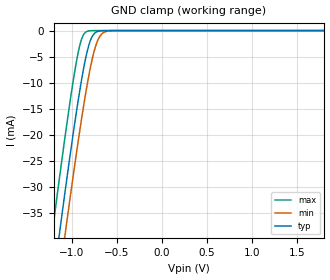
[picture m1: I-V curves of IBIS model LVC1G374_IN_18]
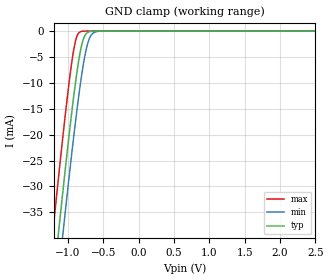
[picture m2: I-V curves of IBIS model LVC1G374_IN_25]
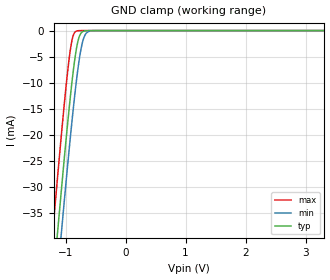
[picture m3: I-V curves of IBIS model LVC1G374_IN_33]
| TEXAS INSTRUMENTS INCORPORATED
| Standard Linear and Logic Group
| IBIS Model of SN74LVC1G374
| Single D-Type Flip-Flop with 3-State Output
| This file contains package information for the following:
|  SOT 6-pin (DBV) package as [Component] LVC1G374_DBV
|  SOT 6-pin (DCK) package as [Component] LVC1G374_DCK
|  DSBGA 6-pin (YEP) package as [Component] LVC1G374_YEP
|  DSBGA 6-pin (YZP) package as [Component] LVC1G374_YZP
| This device can be powered at the following Vccs:
|  1.8 volt Vcc
|  2.5 volt Vcc
|  3.3 volt Vcc
|  5 volt Vcc
| This file provides unique models under the [Model Selector] for each Vcc.
| For operation at a specific Vcc, select the appropriate model after each
| [Model Selector] keyword.
[IBIS Ver]   3.2
[Comment char]  |_char
[File Name]   sn74lvc1g374.ibs
[File Rev]   1.2 | x_die
[Date]   May 27, 2003
[Source]   Data created from TI-SPICE simulations at TI-SLL.
[Notes]   The following is an IBIS list for the LVC1G374.
   Please contact sllibis@ti.com with questions and
   comments concerning SLL IBIS models.
   - FILE REV HISTORY
   - 1.2 YEP and YZP packages released on 05/27/04
   - Due to the fact that the Device is 5.5-V Input tolarent,
   the pulldown model has some Non-Monotonic Warnings.
   - Power clamp data deleted as there is no power-clamp diode.
[Disclaimer] Property of Texas Instruments Incorporated.  Unauthorized
   reproduction and/or distribution is strictly prohibited.
   This product is protected under copyright law.
   Created  2003, (C) Copyright  2003, Texas Instruments
   Incorporated, All Rights Reserved
   UNLESS THERE IS A SIGNED, WRITTEN AGREEMENT TO THE
   CONTRARY, TEXAS INSTRUMENTS (TI) IS PROVIDING THE IBIS
   MODELS  AND WITHOUT ANY WARRANTY, EXPRESSED OR
   IMPLIED.  TI assumes no liability for:
   1) the accuracy of the IBIS models provided to your
   company;
   2) the proper functioning of these IBIS Models in your
   design or for any resulting applications; or
   3) infringement of patents, copyrights or intellectual
   property rights resulting from your use of these IBIS
   models.
   TI provides IBIS Models as a service to our customers.
   You and your company shall not distribute, sell or give
   these models to anyone else without prior written
   permission from TI.
   TI reserves the right to make changes to our products or
   to discontinue any semiconductor product or service
   without notice, and advises our customers to obtain the
   latest version of relevant information to verify, before
   placing orders, that the information being relied on is
   current.
   Please be aware that your receipt and use of the IBIS
   information provided shall serve as acceptance of these
   terms and conditions.  If you do not accept these terms,
   you should return or destroy the IBIS models and any
   other accompanying information immediately.
| Component LVC1G374_DBV 6-pin SOT
[Component]   LVC1G374_DBV
[Manufacturer]   Texas Instruments, Inc.
[Package]
|   typ   min   max
R_pkg   2.500e-02   1.900e-02   3.700e-02
L_pkg   1.524e-09   1.260e-09   1.751e-09
C_pkg   2.450e-13   1.980e-13   2.640e-13
[Pin]   signal_name   model_name   R_pin   L_pin   C_pin
1   CLK   LVC1G374_IN   2.100e-02   1.405e-09   2.460e-13
2   GND   GND   3.700e-02   1.751e-09   2.630e-13
3   D   LVC1G374_IN   2.600e-02   1.493e-09   2.470e-13
4   Q   LVC1G374_OUT   1.900e-02   1.620e-09   2.640e-13
5   VCC   POWER   2.400e-02   1.260e-09   1.980e-13
6   NOE   LVC1G374_IN   2.100e-02   1.617e-09   2.500e-13
| Component LVC1G374_DCK 6-pin SOT
[Component]   LVC1G374_DCK
[Manufacturer]   Texas Instruments, Inc.
[Package]
|   typ   min   max
R_pkg   1.400e-02   1.100e-02   2.100e-02
L_pkg   9.480e-10   7.840e-10   1.103e-09
C_pkg   1.910e-13   1.670e-13   2.050e-13
[Pin]   signal_name   model_name   R_pin   L_pin   C_pin
1   CLK   LVC1G374_IN   1.300e-02   9.840e-10   1.960e-13
2   GND   GND   2.100e-02   1.103e-09   2.050e-13
3   D   LVC1G374_IN   1.100e-02   9.980e-10   1.970e-13
4   Q   LVC1G374_OUT   1.300e-02   9.040e-10   1.900e-13
5   VCC   POWER   1.500e-02   7.840e-10   1.670e-13
6   NOE   LVC1G374_IN   1.200e-02   9.160e-10   1.950e-13
| Component LVC1G374_YEP 6-pin DSBGA
[Component]   LVC1G374_YEP
[Manufacturer]   Texas Instruments, Inc.
[Package]
|   typ   min   max
R_pkg   1.000e-03   1.000e-03   2.100e-02
L_pkg   2.450e-11   2.400e-11   1.103e-09
C_pkg   5.600e-14   0.000e+00   2.050e-13
[Pin]   signal_name   model_name   R_pin   L_pin   C_pin
1   CLK   LVC1G374_IN   1.000e-03   2.500e-11   6.400e-14
2   GND   GND   1.000e-03   2.400e-11   6.700e-14
3   D   LVC1G374_IN   1.000e-03   2.500e-11   6.400e-14
4   Q   LVC1G374_OUT   1.000e-03   2.500e-11   6.400e-14
5   VCC   POWER   1.000e-03   2.400e-11   6.700e-14
6   NOE   LVC1G374_IN   1.000e-03   2.500e-11   6.400e-14
| Component LVC1G374_YZP 6-pin DSBGA
[Component]   LVC1G374_YZP
[Manufacturer]   Texas Instruments, Inc.
[Package]
|   typ   min   max
R_pkg   1.000e-03   1.000e-03   2.100e-02
L_pkg   2.450e-11   2.400e-11   1.103e-09
C_pkg   5.600e-14   0.000e+00   2.050e-13
[Pin]   signal_name   model_name   R_pin   L_pin   C_pin
1   CLK   LVC1G374_IN   1.000e-03   2.500e-11   6.400e-14
2   GND   GND   1.000e-03   2.400e-11   6.700e-14
3   D   LVC1G374_IN   1.000e-03   2.500e-11   6.400e-14
4   Q   LVC1G374_OUT   1.000e-03   2.500e-11   6.400e-14
5   VCC   POWER   1.000e-03   2.400e-11   6.700e-14
6   NOE   LVC1G374_IN   1.000e-03   2.500e-11   6.400e-14
| Model LVC1G374_IN
[Model Selector]   LVC1G374_IN
LVC1G374_IN_18   1.8 volt Vcc
LVC1G374_IN_25   2.5 volt Vcc
LVC1G374_IN_33   3.3 volt Vcc
LVC1G374_IN_50   5 volt Vcc
| Model LVC1G374_OUT
[Model Selector]   LVC1G374_OUT
LVC1G374_OUT_18   1.8 volt Vcc
LVC1G374_OUT_25   2.5 volt Vcc
LVC1G374_OUT_33   3.3 volt Vcc
LVC1G374_OUT_50   5 volt Vcc
| Models and submodels in the file (8): LVC1G374_IN_18 (Input), LVC1G374_IN_25 (Input), LVC1G374_IN_33 (Input), LVC1G374_IN_50 (Input), LVC1G374_OUT_18 (3-state), LVC1G374_OUT_25 (3-state), LVC1G374_OUT_33 (3-state), LVC1G374_OUT_50 (3-state)
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[Model]   LVC1G374_IN_18
Model_type  Input
Vinl=0.5775
Vinh=1.2675
| variable   typ   min   max
C_comp   3.12pF   2.66pF   3.83pF
[Temperature Range]   40   100   -40
| Ambient temperature   25   85   -40
[Voltage range]   1.8   1.65   1.95
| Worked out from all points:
|   GND clamp passes 1 mA (typ) near -0.77 V on its own axis
[GND Clamp]
| LVC1G374_IN_18
|   Voltage   I(typ)   I(min)   I(max)
-5.5V     -655.2mA   -662.2mA   -646.6mA
-1.215V   -49.6mA    -57.88mA   -38.96mA
-1.135V   -39.07mA   -47.36mA   -28.42mA
-1.075V   -31.35mA   -39.6mA    -20.75mA
-1.055V   -28.82mA   -37.05mA   -18.27mA
-955mV    -16.68mA   -24.66mA   -6.874mA
-885mV    -9.098mA   -16.55mA   -1.486mA
-825mV    -3.922mA   -10.26mA   -137.1uA
-780mV    -1.472mA   -6.227mA   -17.15uA
-715mV    -205.4uA   -2.128mA   -808.5nA
-650mV    -22.01uA   -443.9uA   -37.93nA
1.8V      3.326pA    6.142pA    3.026pA
[Model]   LVC1G374_IN_25
Model_type  Input
Vinl=0.7
Vinh=1.7
| variable   typ   min   max
C_comp   3.02pF   2.47pF   3.85pF
[Temperature Range]   40   100   -40
| Ambient temperature   25   85   -40
[Voltage range]   2.5   2.3   2.7
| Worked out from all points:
|   GND clamp passes 1 mA (typ) near -0.77 V on its own axis
[GND Clamp]
| LVC1G374_IN_25
|   Voltage   I(typ)   I(min)   I(max)
-5.5V     -655.2mA   -662.2mA   -646.6mA
-1.215V   -49.6mA    -57.88mA   -38.96mA
-1.14V    -39.72mA   -48.01mA   -29.07mA
-1.12V    -37.12mA   -45.41mA   -26.48mA
-1.08V    -31.98mA   -40.25mA   -21.38mA
-1.06V    -29.44mA   -37.69mA   -18.89mA
-960mV    -17.26mA   -25.26mA   -7.377mA
-890mV    -9.597mA   -17.1mA    -1.734mA
-785mV    -1.671mA   -6.635mA   -21.67uA
-720mV    -242.5uA   -2.354mA   -1.023uA
-650mV    -22.01uA   -443.9uA   -37.93nA
2.5V      4.713pA    7.577pA    4.389pA
[Model]   LVC1G374_IN_33
Model_type  Input
Vinl=0.8
Vinh=2.0
| variable   typ   min   max
C_comp   2.92pF   2.34pF   3.83pF
[Temperature Range]   40   100   -40
| Ambient temperature   25   85   -40
[Voltage range]   3.3   3   3.6
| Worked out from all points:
|   GND clamp passes 1 mA (typ) near -0.77 V on its own axis
[GND Clamp]
| LVC1G374_IN_33
|   Voltage   I(typ)   I(min)   I(max)
-5.5V     -655.2mA   -662.2mA   -646.6mA
-1.225V   -50.93mA   -59.21mA   -40.3mA
-1.145V   -40.37mA   -48.66mA   -29.72mA
-1.12V    -37.12mA   -45.41mA   -26.48mA
-1.08V    -31.98mA   -40.25mA   -21.38mA
-1.06V    -29.44mA   -37.69mA   -18.89mA
-965mV    -17.84mA   -25.87mA   -7.89mA
-885mV    -9.098mA   -16.55mA   -1.486mA
-780mV    -1.472mA   -6.227mA   -17.15uA
-715mV    -205.4uA   -2.128mA   -808.5nA
-640mV    -15.53uA   -338.1uA   -23.69nA
3.3V      6.304pA    9.258pA    5.93pA
